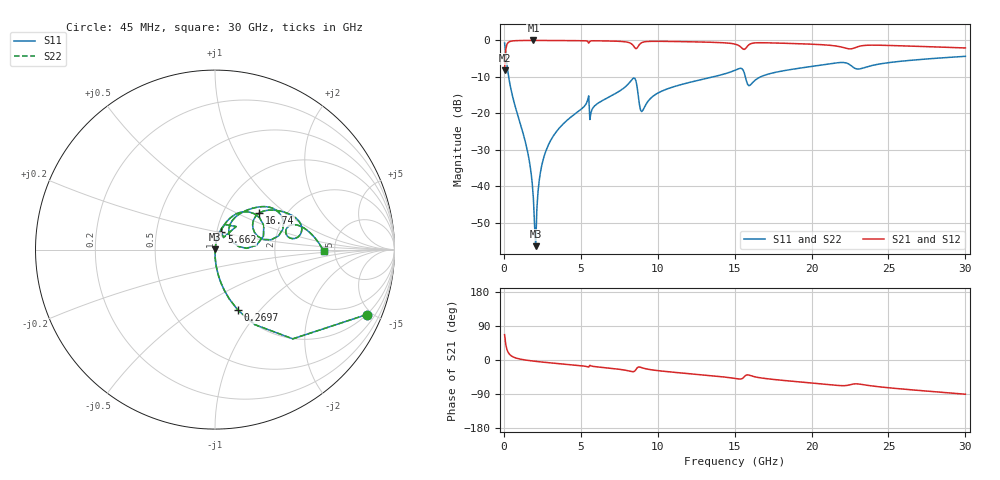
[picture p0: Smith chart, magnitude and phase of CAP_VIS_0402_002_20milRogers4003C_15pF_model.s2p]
! S-parameter model data by Modelithics Inc.  support@modelithics.com  813-866-6335  Tampa FL USA
! S-Parameter data specifications:
! Substrate: 20-mil Rogers 4003C, substrate thickness, H=0.508mm, Dielectric constant, Er=3.75
! PCB Mounting Pad Footprint: Pad width, PadW=0.50mm , Pad length, PadL=0.50mm , Pad gap, PadG (edge-to-edge)=0.40mm , Reference planes=1.4mm apart
! Created Wed Nov 18 12:52:06 2015
# hz S ma R 50
! 2 Port Network Data from SP1.SP block
! freq  magS11  angS11  magS21  angS21  magS12  angS12  magS22  angS22
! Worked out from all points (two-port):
!   401 points, 45 MHz to 30 GHz, reference 50 ohm
!   highest |S21| = -0.01 dB at 1.917 GHz (marker M1); lowest = -8.1 dB at 45 MHz (marker M2)
!   |S21| within 3 dB of the highest: 112.9 MHz to end of sweep
!   lowest |S11| = -56.4 dB at 2.067 GHz (marker M3), VSWR 1.00, Z = 50.1 + j0.102 ohm
!   |S11| at or under -10 dB: 311.1 MHz to 13.58 GHz (13.27 GHz wide, 191 % of centre); 15.7 GHz to 16.68 GHz (976.1 MHz wide, 6.03 % of centre)
!   |S22| runs from -56.4 to -0.7 dB; largest |S21 - S12| = 0
!   S11 on the Smith chart (normalised r, x): 45 MHz: 0.99, -4.68; 269.7 MHz: 0.99, -0.77; 5.662 GHz: 1.05, +0.21; 16.74 GHz: 1.48, +0.67; 30 GHz: 4.07, -0.11
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4.5e7  0.9199 -23.2  0.3921 66.8  0.3921 66.8  0.9199 -23.2
2.696625e8  0.3591 -69.4  0.9329 20.6  0.9329 20.6  0.3591 -69.4
5.692125e8  0.1687 -81.1  0.9851 8.7  0.9851 8.7  0.1687 -81.1
1.54275e9  0.02962 -89.2  0.9986 -1.0  0.9986 -1.0  0.02962 -89.2
1.767412e9  0.01524 -88.5  0.9988 -2.2  0.9988 -2.2  0.01524 -88.5
1.917188e9  0.006809 -84.3  0.9989 -2.9  0.9989 -2.9  0.006809 -84.3
2.066962e9  0.001519 42.0  0.9989 -3.6  0.9989 -3.6  0.001519 42.0
2.4414e9  0.01857 81.2  0.9986 -5.3  0.9986 -5.3  0.01857 81.2
2.890725e9  0.03694 81.0  0.998 -7.1  0.998 -7.1  0.03694 81.0
5.062462e9  0.1161 73.5  0.9907 -15.4  0.9907 -15.4  0.1161 73.5
5.661562e9  0.103 69.7  0.9861 -15.6  0.9861 -15.6  0.103 69.7
8.357512e9  0.2959 42.6  0.8742 -30.8  0.8742 -30.8  0.2959 42.6
8.582175e9  0.2801 15.6  0.7708 -25.3  0.7708 -25.3  0.2801 15.6
8.956612e9  0.106 32.2  0.9315 -20.2  0.9315 -20.2  0.106 32.2
1.007992e10  0.1936 59.0  0.9721 -28.4  0.9721 -28.4  0.1936 59.0
1.50225e10  0.3902 36.7  0.8896 -48.7  0.8896 -48.7  0.3902 36.7
1.577138e10  0.276 11.8  0.8035 -39.6  0.8035 -39.6  0.276 11.8
1.674491e10  0.3211 39.5  0.9297 -47.5  0.9297 -47.5  0.3211 39.5
2.003996e10  0.4415 28.0  0.8872 -60.8  0.8872 -60.8  0.4415 28.0
2.258614e10  0.4487 8.0  0.7677 -64.5  0.7677 -64.5  0.4487 8.0
2.505742e10  0.4974 15.0  0.8531 -73.5  0.8531 -73.5  0.4974 15.0
3e10  0.6055 -0.8  0.7885 -90.3  0.7885 -90.3  0.6055 -0.8
